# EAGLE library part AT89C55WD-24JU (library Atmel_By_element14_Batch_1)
8-bit Microcontroller with 20K Bytes Flash
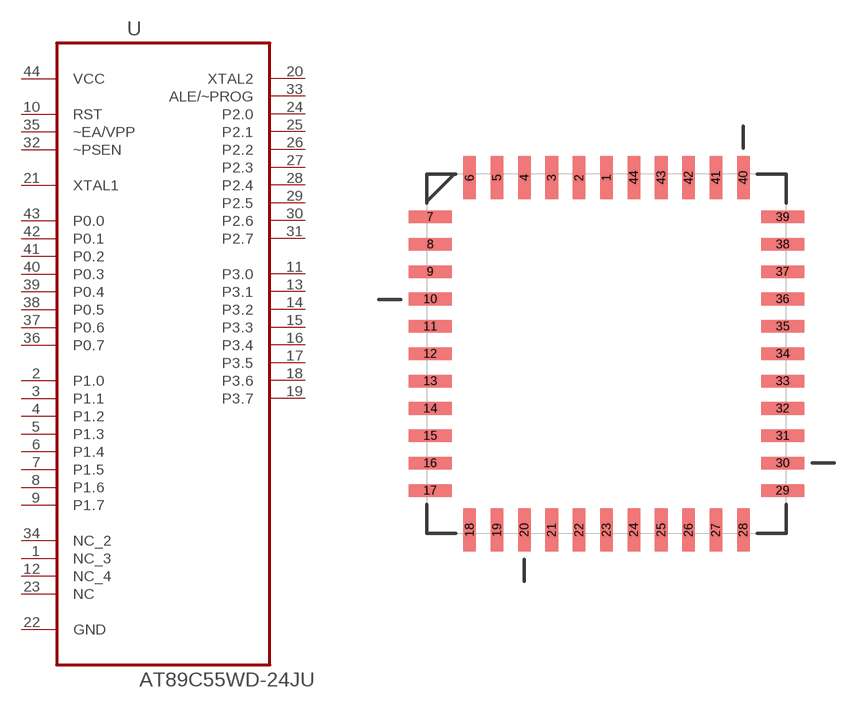
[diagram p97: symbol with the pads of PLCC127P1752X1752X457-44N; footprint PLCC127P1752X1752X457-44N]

Designator prefix U

## AT89C55WD-24JU (MPN: AT89C55WD-24JU; OC_FARNELL: 1095731; OC_NEWARK: 96K6571; PACKAGE: PLCC-44; SUPPLIER: Atmel)  [PLCC127P1752X1752X457-44N]
1  NC_3  nc
2  P1.0
3  P1.1
4  P1.2
5  P1.3
6  P1.4
7  P1.5
8  P1.6
9  P1.7
10  RST  in
11  P3.0
12  NC_4  nc
13  P3.1
14  P3.2
15  P3.3
16  P3.4
17  P3.5
18  P3.6
19  P3.7
20  XTAL2  out
21  XTAL1  in
22  GND  pas
23  NC  nc
24  P2.0
25  P2.1
26  P2.2
27  P2.3
28  P2.4
29  P2.5
30  P2.6
31  P2.7
32  ~PSEN  in
33  ALE/~PROG  out
34  NC_2  nc
35  ~EA/VPP  in
36  P0.7
37  P0.6
38  P0.5
39  P0.4
40  P0.3
41  P0.2
42  P0.1
43  P0.0
44  VCC  pwr

## Footprint PLCC127P1752X1752X457-44N (pad centres in mm)
smd 0.584 x 2.007: 1 0,8.179; 2 -1.27,8.179; 3 -2.54,8.179; 4 -3.81,8.179; 5 -5.08,8.179; 6 -6.35,8.179; 18 -6.35,-8.179; 19 -5.08,-8.179; 20 -3.81,-8.179; 21 -2.54,-8.179; 22 -1.27,-8.179; 23 0,-8.179; 24 1.27,-8.179; 25 2.54,-8.179; 26 3.81,-8.179; 27 5.08,-8.179; 28 6.35,-8.179; 40 6.35,8.179; 41 5.08,8.179; 42 3.81,8.179; 43 2.54,8.179; 44 1.27,8.179
smd 2.007 x 0.584: 7 -8.179,6.35; 8 -8.179,5.08; 9 -8.179,3.81; 10 -8.179,2.54; 11 -8.179,1.27; 12 -8.179,0; 13 -8.179,-1.27; 14 -8.179,-2.54; 15 -8.179,-3.81; 16 -8.179,-5.08; 17 -8.179,-6.35; 29 8.179,-6.35; 30 8.179,-5.08; 31 8.179,-3.81; 32 8.179,-2.54; 33 8.179,-1.27; 34 8.179,0; 35 8.179,1.27; 36 8.179,2.54; 37 8.179,3.81; 38 8.179,5.08; 39 8.179,6.35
